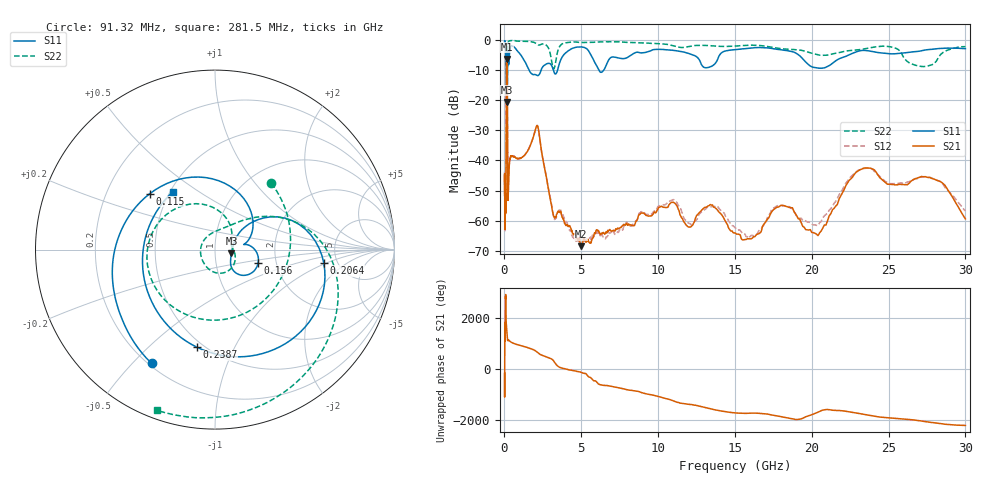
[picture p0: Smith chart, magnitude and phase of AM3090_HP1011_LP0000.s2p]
! Date/Time: Thu, Feb 28, 2019 2:05 PM
! Network Analyzer: Agilent Technologies E8364B Rev: A.07.50.67
! Sweep from 0.010 to 30.000 GHz, 1601 Points, Sweep Type: LOG
! Power Supply: 5.023 V, 0.002 A
# Hz S DB R 50
!freq MagS11 AngS11 MagS21 AngS21 MagS12 AngS12 MagS22 AngS22
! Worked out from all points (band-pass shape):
!   1601 points, 10 MHz to 30 GHz, reference 50 ohm
!   highest |S21| = -6.33 dB at 149.1 MHz (marker M1); lowest = -68.5 dB at 5.002 GHz (marker M2)
!   |S21| within 3 dB of the highest: 128.6 MHz to 177.9 MHz (49.37 MHz wide, 32.2 % of centre)
!   lowest |S11| = -20.6 dB at 181.3 MHz (marker M3), VSWR 1.21, Z = 60 - j2.53 ohm
!   |S11| at or under -10 dB: 1.604 GHz to 2.382 GHz (778.5 MHz wide, 39.1 % of centre); 3.188 GHz to 3.459 GHz (270.7 MHz wide, 8.14 % of centre); 6.145 GHz to 6.464 GHz (319.4 MHz wide, 5.07 % of centre)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
!   |S22| runs from -22.0 to -0.1 dB; largest |S21 - S12| = 0.012
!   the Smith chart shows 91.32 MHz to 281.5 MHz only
!   S11 on the Smith chart (normalised r, x): 91.32 MHz: 0.21, -0.57; 115 MHz: 0.39, +0.32; 156 MHz: 1.61, -0.25; 206.4 MHz: 3.90, -0.91; 238.7 MHz: 0.46, -0.72; 281.5 MHz: 0.52, +0.39
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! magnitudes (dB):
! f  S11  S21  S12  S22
! 10 MHz  -0.3  -45.1  -43.8  -0.5
! 38.04 MHz  -0.4  -59.7  -58.4  -1.2
! 42.47 MHz  -0.6  -61.0  -63.1  -1.5
! 48.85 MHz  -0.7  -48.6  -49.5  -1.3
! 91.32 MHz  -2.8  -57.2  -57.2  -6.3
! 115 MHz  -6.4  -22.9  -22.8  -8.2
! 144.7 MHz  -14.3  -6.4  -6.4  -19.1
! 149.1 MHz  -13.0  -6.3  -6.3  -17.8
! 156 MHz  -12.0  -6.4  -6.4  -17.2
! 181.3 MHz  -20.6  -10.8  -10.8  -16.8
! 206.4 MHz  -4.3  -48.1  -46.6  -2.5
! 238.7 MHz  -5.1  -51.9  -51.2  -0.8
! 281.5 MHz  -8.0  -44.8  -45.2  -0.4
! 550.5 MHz  -2.1  -38.7  -38.6  -0.2
! 2.084 GHz  -11.7  -28.7  -28.6  -1.3
! 3.22 GHz  -10.5  -58.6  -59.1  -9.6
! 5.002 GHz  -2.3  -68.5  -66.0  -0.8
! 7.926 GHz  -6.0  -61.0  -60.7  -0.8
! 10.81 GHz  -3.3  -54.2  -53.4  -1.7
! 20.2 GHz  -9.1  -64.2  -61.4  -4.6
! 23.48 GHz  -3.5  -42.5  -42.7  -2.9
! 30 GHz  -2.8  -59.4  -56.8  -2.2
